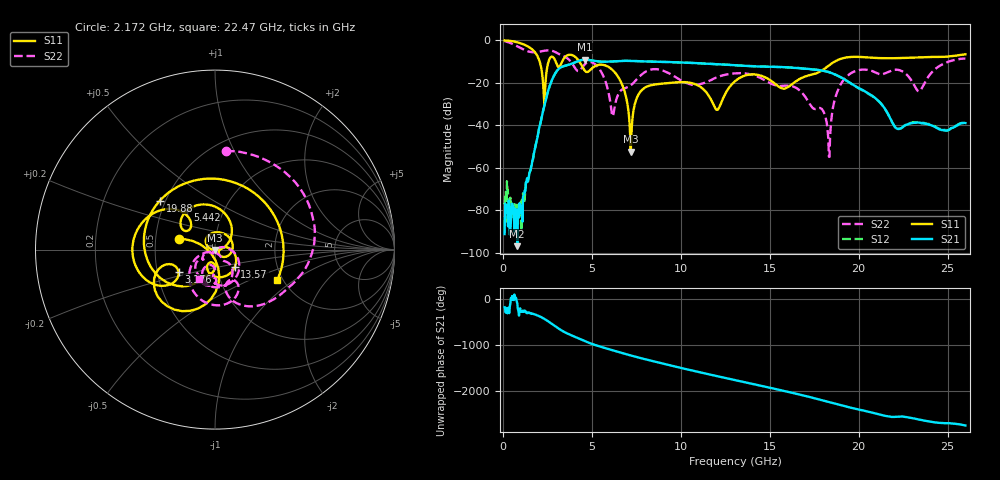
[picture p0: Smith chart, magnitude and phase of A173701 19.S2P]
!  2-Port S-parameters saved by WinCal
! VAR MeasName=S-Parameters (CALIBRATED_DATA) read from VNA (N5245A)
! VAR MeasDate=2017-6-7 10:29:38
! VAR NAME=A173701 19
! VAR FILENAME=A173701 19.S2P
! VAR DATE=2017-6-7 10:29:38
! VAR PHYS_PORTS=1,2
# Hz S DB R 50
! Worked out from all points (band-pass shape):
!   801 points, 100 MHz to 26 GHz, reference 50 ohm
!   highest |S21| = -9.05 dB at 4.633 GHz (marker M1); lowest = -96.9 dB at 812.2 MHz (marker M2)
!   |S21| within 3 dB of the highest: 3.448 GHz to 13.77 GHz (10.32 GHz wide, 120 % of centre)
!   lowest |S11| = -52.4 dB at 7.19 GHz (marker M3), VSWR 1.00, Z = 50 - j0.239 ohm
!   |S11| at or under -10 dB: 2.072 GHz to 2.566 GHz (494.7 MHz wide, 21.3 % of centre); 2.972 GHz to 3.331 GHz (358.7 MHz wide, 11.4 % of centre); 4.302 GHz to 18.65 GHz (14.34 GHz wide, 125 % of centre)
!   |S22| runs from -54.8 to -0.3 dB; largest |S21 - S12| = 0.004
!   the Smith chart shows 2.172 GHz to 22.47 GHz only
!   S11 on the Smith chart (normalised r, x): 2.172 GHz: 0.66, +0.08; 3.176 GHz: 0.64, -0.17; 5.442 GHz: 0.67, +0.32; 13.57 GHz: 1.22, -0.24; 19.88 GHz: 0.47, +0.31; 22.47 GHz: 1.88, -0.74
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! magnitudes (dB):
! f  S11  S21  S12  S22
! 100 MHz  0.0  -91.2  -77.3  -0.3
! 812.2 MHz  -0.9  -96.9  -82.1  -2.8
! 2.172 GHz  -13.6  -36.6  -36.5  -5.1
! 3.176 GHz  -12.5  -13.2  -13.2  -6.5
! 4.438 GHz  -11.9  -9.2  -9.2  -13.0
! 4.633 GHz  -14.5  -9.1  -9.1  -11.0
! 5.442 GHz  -11.4  -10.0  -10.0  -13.6
! 6.186 GHz  -14.1  -9.9  -9.9  -35.7
! 7.19 GHz  -52.4  -9.7  -9.6  -21.1
! 7.676 GHz  -24.8  -9.8  -9.8  -17.0
! 8.744 GHz  -20.5  -10.0  -10.1  -13.6
! 12.05 GHz  -32.7  -11.2  -11.2  -17.3
! 13.05 GHz  -19.2  -11.7  -11.7  -15.5
! 13.57 GHz  -16.7  -11.9  -11.9  -15.5
! 17.39 GHz  -16.1  -13.7  -13.6  -31.5
! 18.33 GHz  -11.8  -15.0  -14.9  -54.7
! 18.85 GHz  -9.2  -16.8  -16.7  -23.2
! 19.88 GHz  -7.7  -21.8  -21.9  -14.2
! 21.69 GHz  -8.4  -35.3  -35.4  -14.7
! 22.47 GHz  -8.3  -40.9  -40.7  -14.6
! 23.41 GHz  -8.0  -38.7  -38.5  -23.9
! 26 GHz  -6.5  -38.9  -38.8  -8.6
